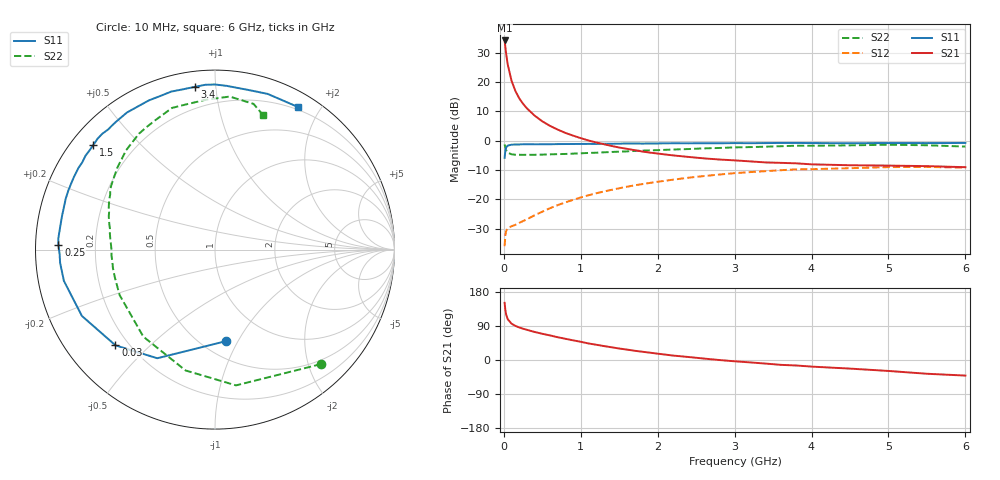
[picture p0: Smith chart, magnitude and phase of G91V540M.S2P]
! SIEMENS Small Signal Semiconductors
! BFG235
! Si NPN RF Bipolar Junction Transistor in SOT223
! VCE = 1.5 V  IC = 40 mA
! Common Emitter S-Parameters:  July  1994
# GHz  S  MA  R  50
!  f  S11  S21  S12  S22
! GHz  MAG  ANG  MAG  ANG  MAG  ANG  MAG  ANG
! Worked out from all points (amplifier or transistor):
!   40 points, 10 MHz to 6 GHz, reference 50 ohm
!   highest |S21| = 34.2 dB at 10 MHz (marker M1)
!   |S21| within 3 dB of that: start of sweep to 23.14 MHz
!   unconditionally stable (mu >= 1): 490.4 MHz to 1.529 GHz
!   at 200 MHz: K = 0.65, MSG = 21.2 dB, |S12| = -28.0 dB
!   at 1.5 GHz: K = 1.01, MAG = 6.4 dB, |S12| = -16.2 dB
!   at 6 GHz: K = 0.95, MSG = 0.1 dB, |S12| = -9.2 dB
!   S11 on the Smith chart (normalised r, x): 10 MHz: 0.65, -0.89; 30 MHz: 0.15, -0.40; 250 MHz: 0.07, +0.01; 1.5 GHz: 0.06, +0.37; 3.4 GHz: 0.08, +0.88; 6 GHz: 0.17, +1.73
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0.01  0.5137 -83.1  51.31 150.8  0.016 62.5  0.8693 -47.2
0.02  0.6855 -118.0  39.35 131.6  0.0249 44.9  0.7655 -81.2
0.03  0.7694 -136.1  30.51 119.8  0.0289 36.2  0.693 -103.7
0.05  0.8286 -153.5  20.11 107.7  0.0321 27.4  0.6281 -129.5
0.1  0.8597 -168.3  10.56 95.9  0.035 25.3  0.5888 -154.5
0.15  0.8661 -175.1  7.08 90.0  0.0369 29.2  0.5791 -164.4
0.2  0.8662 -178.5  5.299 85.9  0.0399 32.8  0.5779 -169.8
0.25  0.8726 178.4  4.268 82.5  0.0429 36.5  0.5758 -173.4
0.3  0.875 175.9  3.571 79.7  0.0459 39.9  0.5773 -176.4
0.4  0.8718 171.4  2.687 74.0  0.0538 44.9  0.5774 179.6
0.5  0.8725 167.7  2.148 69.2  0.0619 48.0  0.5814 176.5
0.6  0.8741 164.6  1.796 64.9  0.071 50.0  0.5872 173.7
0.7  0.8788 161.1  1.553 60.1  0.0801 51.4  0.593 171.1
0.9  0.8819 155.4  1.225 51.9  0.0985 51.5  0.6044 166.8
1.1  0.8864 149.1  1.013 43.7  0.1178 50.6  0.6207 162.4
1.5  0.8945 139.2  0.768 30.3  0.1552 46.1  0.6534 154.1
2.2  0.9078 122.7  0.564 11.7  0.2176 34.7  0.7105 139.9
3.2  0.9107 101.3  0.446 -6.3  0.2927 15.5  0.7812 119.5
3.4  0.9137 97.1  0.428 -9.4  0.3037 11.4  0.7932 115.0
4.5  0.9087 77.9  0.383 -22.7  0.3413 -9.3  0.8364 93.6
5.5  0.9129 65.2  0.37 -36.3  0.3591 -27.2  0.8397 75.2
6  0.9192 59.8  0.355 -41.1  0.3479 -33.9  0.7975 70.5
